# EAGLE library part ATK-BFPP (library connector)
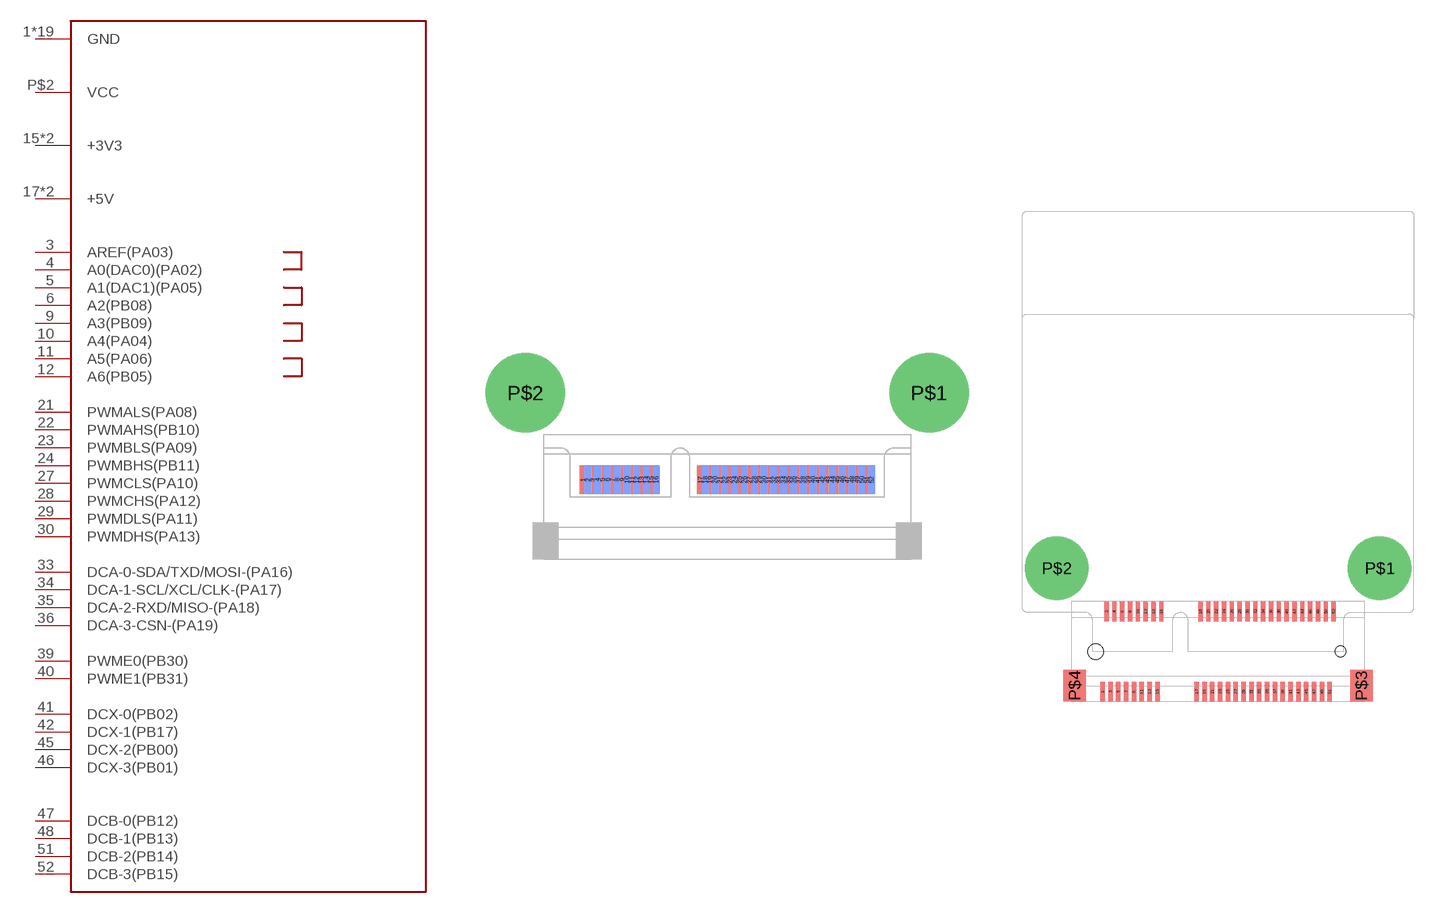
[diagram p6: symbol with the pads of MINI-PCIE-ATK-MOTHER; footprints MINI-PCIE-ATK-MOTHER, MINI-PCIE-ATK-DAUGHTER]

Designator prefix J

## ATK-BFPPMINIPCIE-MOTHER  [MINI-PCIE-ATK-MOTHER]
1  GND
2  GND
3  AREF(PA03)
4  A0(DAC0)(PA02)
5  A1(DAC1)(PA05)
6  A2(PB08)
7  GND
8  GND
9  A3(PB09)
10  A4(PA04)
11  A5(PA06)
12  A6(PB05)
13  GND
14  GND
15  +3V3
16  +3V3
17  +5V
18  +5V
19  GND
20  GND
21  PWMALS(PA08)
22  PWMAHS(PB10)
23  PWMBLS(PA09)
24  PWMBHS(PB11)
25  GND
26  GND
27  PWMCLS(PA10)
28  PWMCHS(PA12)
29  PWMDLS(PA11)
30  PWMDHS(PA13)
31  GND
32  GND
33  DCA-0-SDA/TXD/MOSI-(PA16)
34  DCA-1-SCL/XCL/CLK-(PA17)
35  DCA-2-RXD/MISO-(PA18)
36  DCA-3-CSN-(PA19)
37  GND
38  GND
39  PWME0(PB30)
40  PWME1(PB31)
41  DCX-0(PB02)
42  DCX-1(PB17)
43  GND
44  GND
45  DCX-2(PB00)
46  DCX-3(PB01)
47  DCB-0(PB12)
48  DCB-1(PB13)
49  GND
50  GND
51  DCB-2(PB14)
52  DCB-3(PB15)
P$1  GND
P$2  VCC

## ATK-BFPPMINIPCIE-DAUGHTER  [MINI-PCIE-ATK-DAUGHTER]
Pads as for MINI-PCIE-ATK-MOTHER

## ATK-BFPPFX8-MOTHER  [ATK-BFPP-BOTTOM-FX8-60]
P$1  GND
P$2  AREF(PA03)
P$3  A0(DAC0)(PA02)
P$4  GND
P$5  A1(DAC1)(PA05)
P$6  A2(PB08)
P$7  GND
P$8  A3(PB09)
P$9  A4(PA04)
P$10  GND
P$11  A5(PA06)
P$12  A6(PB05)
P$13  GND
P$14  GND
P$15  PWME0(PB30)
P$16  PWME1(PB31)
P$17  GND
P$18  GND
P$19  DCX-2(PB00)
P$20  DCX-3(PB01)
P$21  GND
P$26  +5V
P$27  +5V
P$28  +3V3
P$29  +3V3
P$30  GND
P$31  GND
P$32  GND
P$33  DCB-3(PB15)
P$34  DCB-2(PB14)
P$35  GND
P$36  DCB-1(PB13)
P$37  DCB-0(PB12)
P$38  GND
P$39  GND
P$40  DCX-1(PB17)
P$41  GND
P$42  DCX-0(PB02)
P$43  GND
P$44  GND
P$45  DCA-3-CSN-(PA19)
P$46  DCA-2-RXD/MISO-(PA18)
P$47  GND
P$48  DCA-1-SCL/XCL/CLK-(PA17)
P$49  DCA-0-SDA/TXD/MOSI-(PA16)
P$50  GND
P$51  GND
P$52  PWMDHS(PA13)
P$53  PWMDLS(PA11)
P$54  PWMCHS(PA12)
P$55  PWMCLS(PA10)
P$56  PWMBHS(PB11)
P$57  PWMBLS(PA09)
P$58  PWMAHS(PB10)
P$59  PWMALS(PA08)
P$60  GND
P$61  VCC
P$62  GND

## ATK-BFPPFX8-DAUGHTER  [ATK-BFPP-TOP-FX8-60]
Pads as for ATK-BFPP-BOTTOM-FX8-60

## ATK-BFPPFX8-THRU  [ATK-BFPP-THRU-FX8-60]
P$1  GND
P$2  AREF(PA03)
P$3  A0(DAC0)(PA02)
P$4  GND
P$5  A1(DAC1)(PA05)
P$6  A2(PB08)
P$7  GND
P$8  A3(PB09)
P$9  A4(PA04)
P$10  GND
P$11  A5(PA06)
P$12  A6(PB05)
P$13  GND
P$14  GND
P$15  PWME0(PB30)
P$16  PWME1(PB31)
P$17  GND
P$18  GND
P$19  DCX-2(PB00)
P$20  DCX-3(PB01)
P$21  GND
P$26  +5V
P$27  +5V
P$28  +3V3
P$29  +3V3
P$30  GND
P$31  GND
P$32  GND
P$33  DCB-3(PB15)
P$34  DCB-2(PB14)
P$35  GND
P$36  DCB-1(PB13)
P$37  DCB-0(PB12)
P$38  GND
P$39  GND
P$40  DCX-1(PB17)
P$41  GND
P$42  DCX-0(PB02)
P$43  GND
P$44  GND
P$45  DCA-3-CSN-(PA19)
P$46  DCA-2-RXD/MISO-(PA18)
P$47  GND
P$48  DCA-1-SCL/XCL/CLK-(PA17)
P$49  DCA-0-SDA/TXD/MOSI-(PA16)
P$50  GND
P$51  GND
P$52  PWMDHS(PA13)
P$53  PWMDLS(PA11)
P$54  PWMCHS(PA12)
P$55  PWMCLS(PA10)
P$56  PWMBHS(PB11)
P$57  PWMBLS(PA09)
P$58  PWMAHS(PB10)
P$59  PWMALS(PA08)
P$60  GND
P$61  VCC
P$62  GND
P$63  GND
P$64  AREF(PA03)
P$65  A0(DAC0)(PA02)
P$66  GND
P$67  A1(DAC1)(PA05)
P$68  A2(PB08)
P$69  GND
P$70  A3(PB09)
P$71  A4(PA04)
P$72  GND
P$73  A5(PA06)
P$74  A6(PB05)
P$75  GND
P$76  GND
P$77  PWME0(PB30)
P$78  PWME1(PB31)
P$79  GND
P$80  GND
P$81  DCX-2(PB00)
P$82  DCX-3(PB01)
P$83  GND
P$88  +5V
P$89  +5V
P$90  +3V3
P$91  +3V3
P$92  GND
P$93  GND
P$94  GND
P$95  DCB-3(PB15)
P$96  DCB-2(PB14)
P$97  GND
P$98  DCB-1(PB13)
P$99  DCB-0(PB12)
P$100  GND
P$101  GND
P$102  DCX-1(PB17)
P$103  GND
P$104  DCX-0(PB02)
P$105  GND
P$106  GND
P$107  DCA-3-CSN-(PA19)
P$108  DCA-2-RXD/MISO-(PA18)
P$109  GND
P$110  DCA-1-SCL/XCL/CLK-(PA17)
P$111  DCA-0-SDA/TXD/MOSI-(PA16)
P$112  GND
P$113  GND
P$114  PWMDHS(PA13)
P$115  PWMDLS(PA11)
P$116  PWMCHS(PA12)
P$117  PWMCLS(PA10)
P$118  PWMBHS(PB11)
P$119  PWMBLS(PA09)
P$120  PWMAHS(PB10)
P$121  PWMALS(PA08)
P$122  GND
P$123  GND
P$124  AREF(PA03)
P$125  A0(DAC0)(PA02)
P$126  GND
P$127  A1(DAC1)(PA05)
P$128  A2(PB08)
P$129  GND
P$130  A3(PB09)
P$131  A4(PA04)
P$132  GND
P$133  A5(PA06)
P$134  A6(PB05)
P$135  GND
P$136  GND
P$137  PWME0(PB30)
P$138  PWME1(PB31)
P$139  GND
P$140  GND
P$141  DCX-2(PB00)
P$142  DCX-3(PB01)
P$143  GND
P$148  +5V
P$149  +5V
P$150  +3V3
P$151  +3V3
P$152  GND
P$153  GND
P$154  GND
P$155  DCB-3(PB15)
P$156  DCB-2(PB14)
P$157  GND
P$158  DCB-1(PB13)
P$159  DCB-0(PB12)
P$160  GND
P$161  GND
P$162  DCX-1(PB17)
P$163  GND
P$164  DCX-0(PB02)
P$165  GND
P$166  GND
P$167  DCA-3-CSN-(PA19)
P$168  DCA-2-RXD/MISO-(PA18)
P$169  GND
P$170  DCA-1-SCL/XCL/CLK-(PA17)
P$171  DCA-0-SDA/TXD/MOSI-(PA16)
P$172  GND
P$173  GND
P$174  PWMDHS(PA13)
P$175  PWMDLS(PA11)
P$176  PWMCHS(PA12)
P$177  PWMCLS(PA10)
P$178  PWMBHS(PB11)
P$179  PWMBLS(PA09)
P$180  PWMAHS(PB10)
P$181  PWMALS(PA08)
P$182  GND

## ATK-BFPP  [ATK-BFPP-0101]
P$A1  +3V3
P$A2  PWME0(PB30)
P$A3  AREF(PA03)
P$A4  GND
P$A5  DCA-2-RXD/MISO-(PA18)
P$A6  DCA-3-CSN-(PA19)
P$A7  GND
P$A8  A3(PB09)
P$A9  A4(PA04)
P$A10  GND
P$B1  +5V
P$B2  PWME1(PB31)
P$B3  A0(DAC0)(PA02)
P$B4  GND
P$B5  DCA-1-SCL/XCL/CLK-(PA17)
P$B6  DCA-0-SDA/TXD/MOSI-(PA16)
P$B7  GND
P$B8  A1(DAC1)(PA05)
P$B9  A5(PA06)
P$B10  GND
P$C1  DCX-2(PB00)
P$C2  DCX-3(PB01)
P$C3  A6(PB05)
P$C4  GND
P$C5  PWMALS(PA08)
P$C6  PWMBLS(PA09)
P$C7  PWMCLS(PA10)
P$C8  PWMDLS(PA11)
P$C9  DCB-2(PB14)
P$C10  DCB-3(PB15)
P$D1  DCX-1(PB17)
P$D2  DCX-0(PB02)
P$D3  A2(PB08)
P$D4  GND
P$D5  PWMAHS(PB10)
P$D6  PWMBHS(PB11)
P$D7  PWMCHS(PA12)
P$D8  PWMDHS(PA13)
P$D9  DCB-1(PB13)
P$D10  DCB-0(PB12)
P$GND  GND
P$VCC  VCC

## Footprint MINI-PCIE-ATK-MOTHER (pad centres in mm)
smd 0.55 x 2.3: 1 -11.8,1.4; 3 -11,1.4; 5 -10.2,1.4; 7 -9.4,1.4; 9 -8.6,1.4; 11 -7.8,1.4; 13 -7,1.4; 15 -6.2,1.4; 17 -2.2,1.4; 19 -1.4,1.4; 21 -0.6,1.4; 23 0.2,1.4; 25 1,1.4; 27 1.8,1.4; 29 2.6,1.4; 31 3.4,1.4; 33 4.2,1.4; 35 5,1.4; 37 5.8,1.4; 39 6.6,1.4; 41 7.4,1.4; 43 8.2,1.4; 45 9,1.4; 47 9.8,1.4; 49 10.6,1.4; 51 11.4,1.4
smd 0.55 x 2.3 bottom: 2 -11.4,1.4; 4 -10.6,1.4; 6 -9.8,1.4; 8 -9,1.4; 10 -8.2,1.4; 12 -7.4,1.4; 14 -6.6,1.4; 16 -5.8,1.4; 18 -1.8,1.4; 20 -1,1.4; 22 -0.2,1.4; 24 0.6,1.4; 26 1.4,1.4; 28 2.2,1.4; 30 3,1.4; 32 3.8,1.4; 34 4.6,1.4; 36 5.4,1.4; 38 6.2,1.4; 40 7,1.4; 42 7.8,1.4; 44 8.6,1.4; 46 9.4,1.4; 48 10.2,1.4; 50 11,1.4; 52 11.8,1.4
drill 4.5 pad 6.5: P$1 16.5,8.5; P$2 -16.5,8.5

## Footprint MINI-PCIE-ATK-DAUGHTER (pad centres in mm)
smd 0.45 x 2: 1 -11.8,-4.1; 2 -11.4,4.1; 3 -11,-4.1; 4 -10.6,4.1; 5 -10.2,-4.1; 6 -9.8,4.1; 7 -9.4,-4.1; 8 -9,4.1; 9 -8.6,-4.1; 10 -8.2,4.1; 11 -7.8,-4.1; 12 -7.4,4.1; 13 -7,-4.1; 14 -6.6,4.1; 15 -6.2,-4.1; 16 -5.8,4.1; 17 -2.2,-4.1; 18 -1.8,4.1; 19 -1.4,-4.1; 20 -1,4.1; 21 -0.6,-4.1; 22 -0.2,4.1; 23 0.2,-4.1; 24 0.6,4.1; 25 1,-4.1; 26 1.4,4.1; 27 1.8,-4.1; 28 2.2,4.1; 29 2.6,-4.1; 30 3,4.1; 31 3.4,-4.1; 32 3.8,4.1; 33 4.2,-4.1; 34 4.6,4.1; 35 5,-4.1; 36 5.4,4.1; 37 5.8,-4.1; 38 6.2,4.1; 39 6.6,-4.1; 40 7,4.1; 41 7.4,-4.1; 42 7.8,4.1; 43 8.2,-4.1; 44 8.6,4.1; 45 9,-4.1; 46 9.4,4.1; 47 9.8,-4.1; 48 10.2,4.1; 49 10.6,-4.1; 50 11,4.1; 51 11.4,-4.1; 52 11.8,4.1
drill 4.5 pad 6.5: P$1 16.5,8.5; P$2 -16.5,8.5
smd 2.3 x 3.2: P$3 14.65,-3.5; P$4 -14.65,-3.5
hole 1.6 at -12.5,0
hole 1.1 at 12.5,0

## Footprint ATK-BFPP-BOTTOM-FX8-60 (pad centres in mm)
smd 0.35 x 1.7 bottom: P$1 -8.7,-2.85; P$2 -8.1,-2.85; P$3 -7.5,-2.85; P$4 -6.9,-2.85; P$5 -6.3,-2.85; P$6 -5.7,-2.85; P$7 -5.1,-2.85; P$8 -4.5,-2.85; P$9 -3.9,-2.85; P$10 -3.3,-2.85; P$11 -2.7,-2.85; P$12 -2.1,-2.85; P$13 -1.5,-2.85; P$14 -0.9,-2.85; P$15 -0.3,-2.85; P$16 0.3,-2.85; P$17 0.9,-2.85; P$18 1.5,-2.85; P$19 2.1,-2.85; P$20 2.7,-2.85; P$21 3.3,-2.85; P$22 3.9,-2.85; P$23 4.5,-2.85; P$24 5.1,-2.85; P$25 5.7,-2.85; P$26 6.3,-2.85; P$27 6.9,-2.85; P$28 7.5,-2.85; P$29 8.1,-2.85; P$30 8.7,-2.85; P$31 8.7,2.85; P$32 8.1,2.85; P$33 7.5,2.85; P$34 6.9,2.85; P$35 6.3,2.85; P$36 5.7,2.85; P$37 5.1,2.85; P$38 4.5,2.85; P$39 3.9,2.85; P$40 3.3,2.85; P$41 2.7,2.85; P$42 2.1,2.85; P$43 1.5,2.85; P$44 0.9,2.85; P$45 0.3,2.85; P$46 -0.3,2.85; P$47 -0.9,2.85; P$48 -1.5,2.85; P$49 -2.1,2.85; P$50 -2.7,2.85; P$51 -3.3,2.85; P$52 -3.9,2.85; P$53 -4.5,2.85; P$54 -5.1,2.85; P$55 -5.7,2.85; P$56 -6.3,2.85; P$57 -6.9,2.85; P$58 -7.5,2.85; P$59 -8.1,2.85; P$60 -8.7,2.85
drill 3.5 pad 6: P$61 -16.5,0; P$62 16.5,0
hole 1.1 at -11.1,-1.8
hole 0.7 at 11.1,-1.8

## Footprint ATK-BFPP-TOP-FX8-60 (pad centres in mm)
smd 0.35 x 1.7: P$1 -8.7,-2.7; P$2 -8.1,-2.7; P$3 -7.5,-2.7; P$4 -6.9,-2.7; P$5 -6.3,-2.7; P$6 -5.7,-2.7; P$7 -5.1,-2.7; P$8 -4.5,-2.7; P$9 -3.9,-2.7; P$10 -3.3,-2.7; P$11 -2.7,-2.7; P$12 -2.1,-2.7; P$13 -1.5,-2.7; P$14 -0.9,-2.7; P$15 -0.3,-2.7; P$16 0.3,-2.7; P$17 0.9,-2.7; P$18 1.5,-2.7; P$19 2.1,-2.7; P$20 2.7,-2.7; P$21 3.3,-2.7; P$22 3.9,-2.7; P$23 4.5,-2.7; P$24 5.1,-2.7; P$25 5.7,-2.7; P$26 6.3,-2.7; P$27 6.9,-2.7; P$28 7.5,-2.7; P$29 8.1,-2.7; P$30 8.7,-2.7; P$31 8.7,2.7; P$32 8.1,2.7; P$33 7.5,2.7; P$34 6.9,2.7; P$35 6.3,2.7; P$36 5.7,2.7; P$37 5.1,2.7; P$38 4.5,2.7; P$39 3.9,2.7; P$40 3.3,2.7; P$41 2.7,2.7; P$42 2.1,2.7; P$43 1.5,2.7; P$44 0.9,2.7; P$45 0.3,2.7; P$46 -0.3,2.7; P$47 -0.9,2.7; P$48 -1.5,2.7; P$49 -2.1,2.7; P$50 -2.7,2.7; P$51 -3.3,2.7; P$52 -3.9,2.7; P$53 -4.5,2.7; P$54 -5.1,2.7; P$55 -5.7,2.7; P$56 -6.3,2.7; P$57 -6.9,2.7; P$58 -7.5,2.7; P$59 -8.1,2.7; P$60 -8.7,2.7
drill 4.5 pad 6.5: P$61 -16.5,0; P$62 16.5,0
hole 1.1 at -11.1,-1.8
hole 0.7 at 11.1,-1.8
